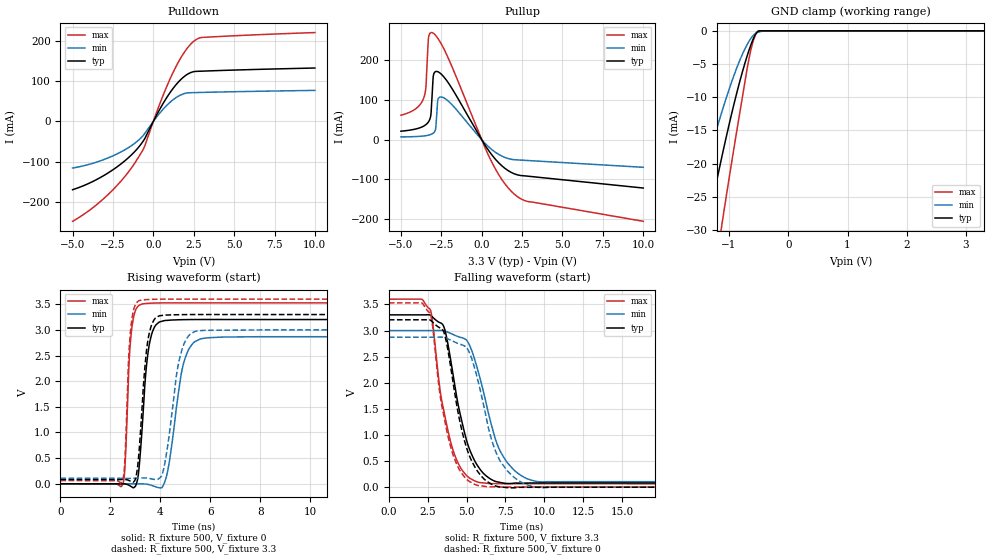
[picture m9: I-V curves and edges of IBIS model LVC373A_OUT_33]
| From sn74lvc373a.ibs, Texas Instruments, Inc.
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[Model]   LVC373A_OUT_33
Model_type  3-state
Enable   Active-Low
Vref =   0
Rref =   500
Cref =   50p
Vmeas =   1.5
| variable   typ   min   max
C_comp   3.11pF   2.87pF   3.41pF
| C_pullup   5.67pF   3.15pF   8.23pF
| C_pulldown   5.76pF   2.89pF   8.17pF
| C_tri-state   3.11pF   2.87pF   3.41pF
[Temperature Range]   40   100   -40
| Ambient temperature   25   85   -40
[Voltage range]   3.3   3   3.6
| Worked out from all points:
|   slope of the pulldown table from 0 to 0.495 V, typ, clamps not added: 13.4 ohm
|   slope of the pullup table from 0 to 0.495 V, typ, clamps not added: 16 ohm
|   GND clamp passes 1 mA (typ) near -0.58 V on its own axis
|   rising waveform, R_fixture 500, V_fixture 0: 20-80 % time 304ps typ, 497ps min, 192ps max; typ from 0 V to 3.2 V
|   falling waveform, R_fixture 500, V_fixture 3.3: 20-80 % time 1.34ns typ, 1.63ns min, 1.15ns max; typ from 3.3 V to 0.082 V
|   rising waveform, R_fixture 500, V_fixture 3.3: 20-80 % time 298ps typ, 485ps min, 182ps max; typ from 0.082 V to 3.3 V
|   falling waveform, R_fixture 500, V_fixture 0: 20-80 % time 1.3ns typ, 1.53ns min, 1.13ns max; typ from 3.21 V to 0 V
[GND Clamp]
| LVC373A_OUT_33
|   Voltage   I(typ)   I(min)   I(max)
-5V       -227.5mA   -167.1mA   -315.1mA
-1.65V    -42.73mA   -29.36mA   -62.5mA
-1.595V   -40.1mA    -27.43mA   -58.85mA
-1.35V    -28.79mA   -19.21mA   -43.1mA
-1.13V    -19.33mA   -12.45mA   -29.74mA
-1.085V   -17.5mA    -11.16mA   -27.11mA
-885mV    -9.904mA   -5.95mA    -15.94mA
-675mV    -3.249mA   -1.766mA   -4.744mA
-630mV    -2.089mA   -1.133mA   -2.824mA
-585mV    -1.089mA   -639uA     -1.35mA
-510mV    -72.18uA   -220.9uA   -61.37uA
3.3V      21.41pA    24.26nA    8.622pA
[Pulldown]
| LVC373A_OUT_33
|   Voltage   I(typ)   I(min)   I(max)
-5V       -169.4mA   -115.6mA   -247.8mA
-3.96V    -153.1mA   -106.4mA   -220.7mA
-2.935V   -131.1mA   -92.67mA   -186.5mA
-1.99V    -105.1mA   -75.42mA   -147.4mA
-1.2V     -76.84mA   -55.78mA   -106.5mA
-565mV    -44.97mA   -31.73mA   -64.05mA
470mV     35.24mA    24.06mA    51.04mA
1.265V    84.07mA    55.04mA    125.1mA
1.93V     111.9mA    69.18mA    172.2mA
2.535V    123.7mA    71.47mA    199.9mA
3.01V     124.7mA    71.95mA    208.2mA
10V       132.5mA    76.94mA    220.4mA
[Pullup]
| LVC373A_OUT_33
|   Voltage   I(typ)   I(min)   I(max)
-5V       21.44mA    6.977mA    61.59mA
-3.6V     34.06mA    9.452mA    103.8mA
-3.455V   37.98mA    10.25mA    132.1mA
-3.29V    45.32mA    11.57mA    257.3mA
-3.145V   63.21mA    13.38mA    269.3mA
-3.045V   130.3mA    15.35mA    268.9mA
-2.855V   171.4mA    26.9mA     262.5mA
-2.71V    170.9mA    100.8mA    254.7mA
-2.435V   162.2mA    106.9mA    236mA
505mV     -31.51mA   -20.64mA   -46.57mA
1.99V     -85.32mA   -50.23mA   -136mA
10V       -121.5mA   -69.39mA   -205.2mA
[Ramp]
| LVC373A_OUT_33
| variable   typ   min   max
dV/dt_r   1.97/3.15E-10   1.77/5.38E-10   2.15/1.98E-10
dV/dt_f   1.93/1.36E-09   1.74/1.67E-09   2.12/1.16E-09
R_load = 500
[Rising Waveform]
| LVC373A_OUT_33
R_fixture =   500
C_fixture =   0
L_fixture =   0
V_fixture =   0
V_fixture_min = 0
V_fixture_max = 0
|   Time   V(typ)   V(min)   V(max)
0s        205.5pV    4.072nV    151.4pV
2.495ns   -467.5uV   -689.9uV   -7.315mV
2.85ns    -59.69mV   -2.218mV   3.008V
3.095ns   99.5mV     -1.284mV   3.456V
3.305ns   1.35V      -1.805mV   3.509V
3.795ns   3.081V     -56.7mV    3.525V
4.255ns   3.186V     165.5mV    3.527V
4.985ns   3.2V       2.441V     3.527V
5.9ns     3.203V     2.847V     3.527V
50ns      3.203V     2.867V     3.527V
[Falling Waveform]
| LVC373A_OUT_33
R_fixture =   500
C_fixture =   0
L_fixture =   0
V_fixture =   3.3
V_fixture_min = 3
V_fixture_max = 3.6
|   Time   V(typ)   V(min)   V(max)
0s        3.3V       3V         3.6V
2.13ns    3.3V       3V         3.598V
2.675ns   3.292V     3V         3.394V
3.51ns    3.094V     2.998V     1.512V
4.47ns    1.567V     2.882V     454.7mV
5.12ns    785.6mV    2.762V     192mV
5.79ns    377.4mV    2.172V     93.55mV
7.215ns   88.3mV     663.1mV    66.88mV
9.545ns   81.46mV    109.7mV    67.06mV
50ns      81.92mV    106.6mV    62.6mV
[Rising Waveform]
| LVC373A_OUT_33
R_fixture =   500
C_fixture =   0
L_fixture =   0
V_fixture =   3.3
V_fixture_min = 3
V_fixture_max = 3.6
|   Time   V(typ)   V(min)   V(max)
0s        81.82mV    106.5mV    62.59mV
2.475ns   83.93mV    106mV      56.65mV
2.82ns    47.2mV     105.7mV    3.054V
3.065ns   247.5mV    109mV      3.537V
3.275ns   1.543V     113.1mV    3.585V
3.745ns   3.196V     85.93mV    3.597V
4.145ns   3.288V     318.4mV    3.6V
4.86ns    3.298V     2.607V     3.6V
5.47ns    3.3V       2.981V     3.6V
50ns      3.3V       3V         3.6V
[Falling Waveform]
| LVC373A_OUT_33
R_fixture =   500
C_fixture =   0
L_fixture =   0
V_fixture =   0
V_fixture_min = 0
V_fixture_max = 0
|   Time   V(typ)   V(min)   V(max)
0s        3.206V     2.872V     3.529V
2.675ns   3.198V     2.872V     3.319V
3.505ns   2.994V     2.87V      1.422V
4.09ns    2.093V     2.801V     659.7mV
4.755ns   1.02V      2.721V     240.8mV
5.745ns   290.1mV    2.028V     32.48mV
6.52ns    73.38mV    1.007V     7.241mV
7.125ns   7.339mV    523.3mV    4.398mV
9.515ns   -449.8uV   2.346mV    4.409mV
50ns      91.94uV    50.74uV    17.11uV
